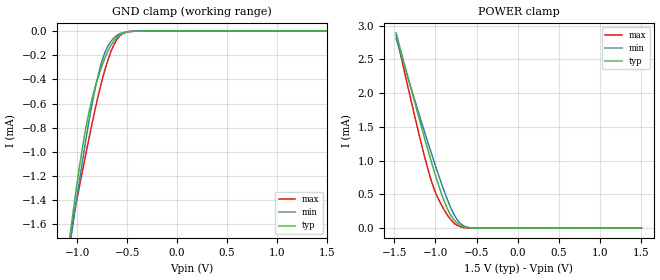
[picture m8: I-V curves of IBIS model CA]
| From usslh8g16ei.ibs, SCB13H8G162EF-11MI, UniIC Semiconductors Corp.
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|   Model CA
[Model] CA
Model_type Input
Polarity   Non-Inverting
Enable   Active-High
Vinl =  0.615V
Vinh =  0.885V
C_comp   88.779fF   72.776fF   0.105pF
C_comp_power_clamp   48.701fF   40.796fF   55.655fF
C_comp_gnd_clamp   40.078fF   31.980fF   49.323fF
[Model Spec]
Vinh   0.885V   0.776V   0.922V
Vinl   0.615V   0.506V   0.652V
[Temperature Range]   45.000   95.000   -40.000
[Voltage Range]   1.500V   1.283V   1.575V
[C Comp Corner]
C_comp_power_clamp   48.701fF   40.796fF   55.655fF
C_comp_gnd_clamp   40.078fF   31.980fF   49.323fF
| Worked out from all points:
|   GND clamp passes 1 mA (typ) near -0.95 V on its own axis
|   POWER clamp passes 1 mA (typ) near -1.05 V on its own axis
[GND_clamp]
|Voltage   I(typ)   I(min)   I(max)
-1.5V     -4.711mA   -4.355mA   -5.13mA
-1.066V   -1.656mA   -1.736mA   -1.672mA
-1.035V   -1.461mA   -1.559mA   -1.532mA
-942mV    -937.4uA   -1.048mA   -1.135mA
-849mV    -553.6uA   -594.1uA   -756.1uA
-787mV    -372.4uA   -351.5uA   -524.2uA
-725mV    -228.7uA   -182.7uA   -326uA
-663mV    -119.4uA   -85.26uA   -170.5uA
-601mV    -49.82uA   -34.44uA   -66.38uA
-539mV    -16.69uA   -11.31uA   -17.4uA
-446mV    -2.392uA   -1.689uA   -1.297uA
1.5V      0A         0A         0A
[POWER_clamp]
|Voltage   I(typ)   I(min)   I(max)
-1.476V   2.894mA    2.812mA    2.865mA
-1.197V   1.625mA    1.687mA    1.386mA
-1.104V   1.219mA    1.323mA    935.8uA
-1.042V   957.4uA    1.086mA    675.5uA
-980mV    709.1uA    854.8uA    475.2uA
-887mV    381.5uA    528.9uA    259.3uA
-825mV    216.9uA    335.6uA    144.5uA
-763mV    108.7uA    177.7uA    64.17uA
-732mV    72.5uA     118.4uA    39.23uA
-670mV    26.52uA    43.96uA    12.12uA
-546mV    1.464uA    3.136uA    422.4nA
1.5V      0A         0A         0A
